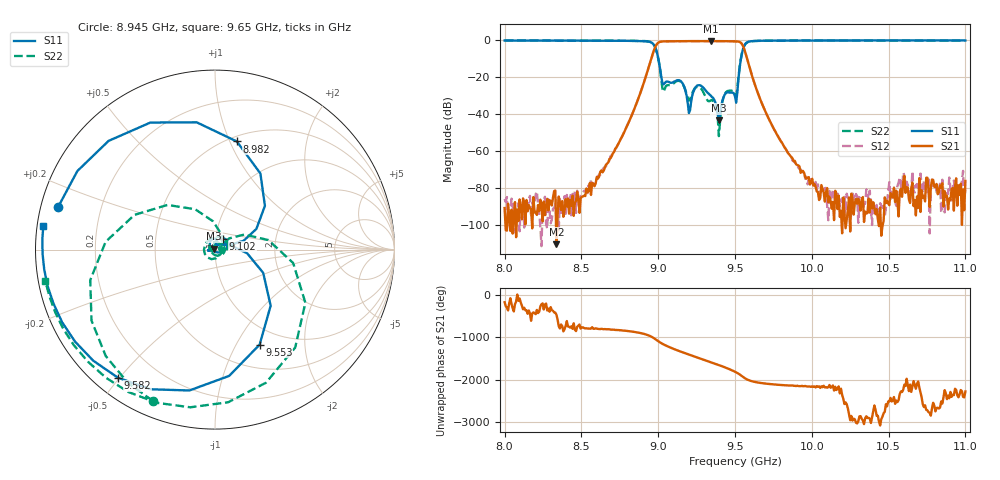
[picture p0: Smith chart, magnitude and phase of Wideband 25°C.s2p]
!Agilent Technologies,N5230C,MY49001174,A.09.42.22
!Agilent N5230C: A.09.42.22
!Date: Friday, February 13, 2026 11:19:52
!Correction: S11(Full 2 Port(1,2))
!S21(Full 2 Port(1,2))
!S12(Full 2 Port(1,2))
!S22(Full 2 Port(1,2))
!S2P File: Measurements: S11, S21, S12, S22:
# Hz S  dB  R 50
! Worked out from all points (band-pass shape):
!   401 points, 8 GHz to 11 GHz, reference 50 ohm
!   highest |S21| = -0.45 dB at 9.342 GHz (marker M1); lowest = -110.4 dB at 8.338 GHz (marker M2)
!   |S21| within 3 dB of the highest: 8.982 GHz to 9.554 GHz (571.9 MHz wide, 6.17 % of centre)
!   lowest |S11| = -43.3 dB at 9.395 GHz (marker M3), VSWR 1.01, Z = 49.6 + j0.526 ohm
!   |S11| at or under -10 dB: 9.001 GHz to 9.539 GHz (537.9 MHz wide, 5.8 % of centre)
!   |S22| runs from -51.9 to -0.1 dB; largest |S21 - S12| = 0.0024
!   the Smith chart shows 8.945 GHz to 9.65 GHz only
!   S11 on the Smith chart (normalised r, x): 8.945 GHz: 0.05, +0.13; 8.982 GHz: 0.55, +1.06; 9.102 GHz: 1.08, +0.13; 9.553 GHz: 0.78, -1.25; 9.582 GHz: 0.07, -0.50; 9.65 GHz: 0.02, +0.07
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8e9  -0.13 73.9  -90.76 -173.9  -85.82 -13.1  -0.14 87.1
8.3375e9  -0.15 42.5  -110.35 -109.6  -90.01 81.9  -0.15 57.6
8.5025e9  -0.17 20.9  -84.71 -48.2  -82.75 -48.6  -0.17 38.7
8.8475e9  -0.37 -85.9  -36.56 -154.9  -36.58 -154.8  -0.29 -39.0
8.945e9  -0.86 164.7  -12.61 113.1  -12.60 113.1  -0.81 -112.4
8.9825e9  -4.23 78.6  -3.35 33.2  -3.35 33.2  -4.28 175.9
9.005e9  -11.79 26.5  -1.07 -24.7  -1.07 -24.7  -12.03 116.1
9.0425e9  -23.21 59.7  -0.60 -101.4  -0.60 -101.4  -26.30 -82.8
9.1025e9  -22.42 54.5  -0.52 163.7  -0.52 163.7  -23.20 93.4
9.1625e9  -23.87 4.4  -0.48 81.5  -0.49 81.5  -24.09 -6.9
9.2225e9  -29.57 146.0  -0.46 4.5  -0.45 4.5  -28.39 33.2
9.29e9  -25.32 79.8  -0.45 -79.5  -0.46 -79.4  -27.51 -50.7
9.3425e9  -29.94 82.5  -0.45 -145.2  -0.45 -145.2  -32.56 152.0
9.395e9  -43.30 129.1  -0.47 146.6  -0.47 146.6  -51.86 -5.4
9.4475e9  -28.22 -175.7  -0.51 73.2  -0.51 73.2  -27.63 125.6
9.5e9  -30.35 168.9  -0.59 -11.5  -0.59 -11.5  -28.87 -7.0
9.5525e9  -4.66 -64.9  -3.14 -133.3  -3.14 -133.3  -4.67 -30.5
9.5825e9  -0.96 -127.1  -11.11 160.5  -11.11 160.5  -1.02 -98.9
9.65e9  -0.30 172.2  -28.83 94.1  -28.83 94.2  -0.34 -169.4
1.00025e10  -0.13 86.8  -74.94 3.4  -76.45 -5.5  -0.15 91.5
1.0505e10  -0.11 41.0  -89.23 10.6  -76.70 -74.5  -0.13 41.7
1.1e10  -0.12 9.8  -76.11 -116.2  -80.79 81.8  -0.15 8.8
